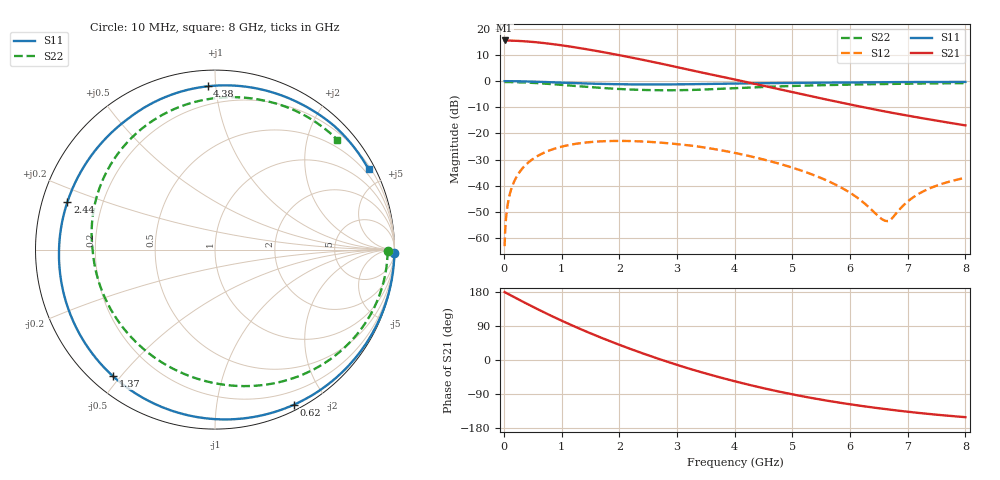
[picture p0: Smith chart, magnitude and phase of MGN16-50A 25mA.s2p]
! Port[1] = GATE
! Port[2] = DRAIN
! [Type]  S-parameter s2p file touchstone ver. 1.0
! [Object]  MGN16-50A
! [Bias]  25 mA
! [Version]  1.0
! [Date]  Thu May 28 10:54:03 2026
! [Source]  This file was created in JSC "ICC Milandr".
! [Disclaimer] Property of JSC "ICC Milandr". Unauthorized reproduction and/or distribution is strictly prohibited.
!  The file and the data are provided "AS IS" and with all faults and disclaim all warranties, express and implied, including
!  without limitation any implied warranties of merchantability, fitness for a particular purpose.
!  JSC "ICC Milandr" assumes no liability for:
!  1) the accuracy of the data provided;
!  2) the proper functioning of this data;
!  3) infringement of patents, copyrights or intellectual property rights resulting from the use of this data.
!  JSC "ICC Milandr" reserves the right to make changes to the products and the data without prior notice.
!  Please, be aware that your receipt and use of the file provided shall serve as acceptance of these terms and conditions.
!  If you do not accept these terms, you should return or destroy this file and any other accompanying information immediately.
# hz S ma R 12.5
! 2 Port Network Data from SP1.SP block
! freq  magS11  angS11  magS21  angS21  magS12  angS12  magS22  angS22
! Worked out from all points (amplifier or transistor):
!   800 points, 10 MHz to 8 GHz, reference 12.5 ohm
!   highest |S21| = 15.6 dB at 10 MHz (marker M1)
!   |S21| within 3 dB of that: start of sweep to 1.336 GHz
!   unconditionally stable (mu >= 1): 4.293 GHz to end of sweep
!   at 1.34 GHz: K = 0.18, MSG = 18.1 dB, |S12| = -23.7 dB
!   at 4.01 GHz: K = 0.86, MSG = 14.0 dB, |S12| = -27.5 dB
!   at 8 GHz: K = 2.50, MAG = 3.2 dB, |S12| = -37.0 dB
!   S11 on the Smith chart (normalised r, x): 10 MHz: open; 620 MHz: 0.06, -1.63; 1.37 GHz: 0.06, -0.48; 2.44 GHz: 0.07, +0.16; 4.38 GHz: 0.09, +0.95; 8 GHz: 0.30, +4.06
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1e7  0.9997 -1.0  5.997 179.2  0.0006992 82.9  0.9618 -0.6
8e7  0.9991 -8.4  5.976 173.5  0.005529 83.0  0.9608 -4.7
1.8e8  0.9966 -18.9  5.928 165.5  0.01234 75.8  0.9567 -10.5
4.1e8  0.9852 -42.4  5.727 147.3  0.02716 58.8  0.9373 -23.6
6.2e8  0.9696 -63.1  5.456 131.3  0.03912 43.6  0.9101 -35.2
7.9e8  0.955 -79.2  5.194 118.7  0.04745 31.7  0.8838 -44.4
9.6e8  0.9398 -94.7  4.909 106.5  0.05447 20.2  0.8556 -53.4
1.14e9  0.9241 -110.3  4.593 94.0  0.06049 8.4  0.8252 -62.8
1.35e9  0.9073 -127.4  4.22 80.0  0.06575 -4.8  0.7909 -73.6
1.37e9  0.9058 -129.0  4.185 78.7  0.06616 -6.1  0.7878 -74.6
1.62e9  0.8894 -147.7  3.751 62.8  0.07 -21.1  0.7513 -87.4
1.87e9  0.8771 -164.8  3.339 47.7  0.07176 -35.4  0.7207 -100.4
2.14e9  0.8685 178.5  2.926 32.1  0.07174 -50.1  0.6954 -114.7
2.44e9  0.8641 162.1  2.511 15.6  0.06984 -65.7  0.6773 -131.0
2.68e9  0.8641 150.3  2.211 3.1  0.06721 -77.6  0.6704 -144.3
3.27e9  0.8737 125.9  1.592 -25.5  0.05798 -105.1  0.679 -176.5
4.01e9  0.8999 102.6  1.07 -56.5  0.04224 -131.4  0.7361 148.2
4.38e9  0.9107 92.6  0.8716 -70.2  0.03427 -142.7  0.7656 132.7
5.34e9  0.9323 70.3  0.5105 -100.4  0.01646 -165.5  0.8279 99.1
6.67e9  0.9568 46.4  0.2547 -130.6  0.002119 -106.0  0.8846 65.7
7.21e9  0.9611 38.4  0.1993 -140.0  0.00721 -53.8  0.9005 55.3
8e9  0.9662 27.6  0.1426 -150.8  0.0142 -58.3  0.9165 41.9
